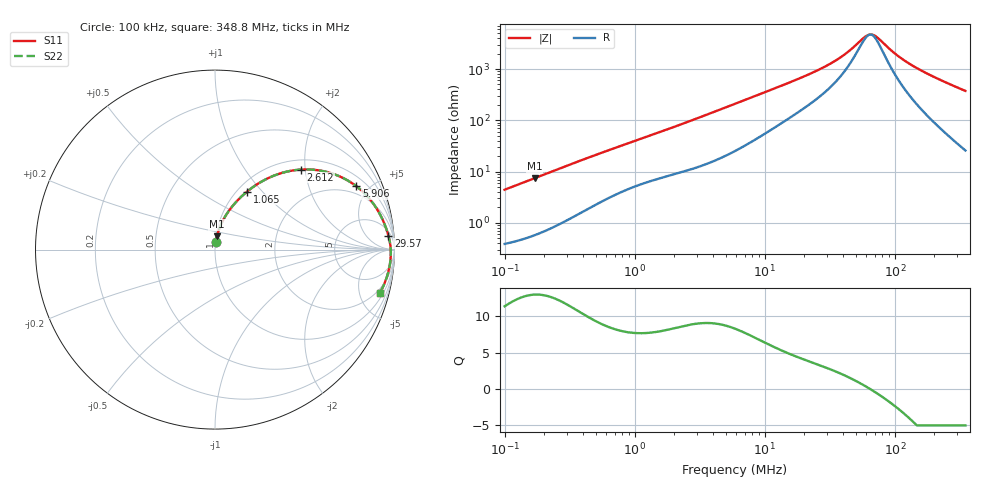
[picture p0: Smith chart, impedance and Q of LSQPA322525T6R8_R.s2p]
! LSQPA322525T6R8_R  S-PARAMETER MODEL  ( General Type )
! Model Generated by TAIYO YUDEN Corporation (http://www.ty-top.com)
! Version 3.0
! TAIYO YUDEN Control No. 110926NF25SB-FKC
! Copyright(c) 2007 TAIYO YUDEN CO.,LTD. All Rights Reserved.
! Product Description (link to TY-COMPAS)
! https://ds.yuden.co.jp/TYCOMPAS/or/detail?pn=LSQPA322525T6R8MR&u=M
! Products Name : Inductors
! Characteristics :
!  Inductance : 6.8 uH , SRF(min) : 50 MHz , DC Resistance(max) : 0.156 Ohm
!  Rated Current : Saturation :950 mA , Temp Rise : 940 mA (40 degC)
!  Case Size : 3.2 x 2.5 / 0.126 x 0.098 [mm/inch] , Thickness : 2.5 / 0.098 [mm/inch]
!  (Conditions: Temperature = 25 degC , DC Bias Current/Voltage = 0A / 0V)
! External Node Assignments :
!  1  o---GGG---o  2
! GND o---------o GND
! Frequency Range : 0.1MHz  -  348.750116MHz  [ 402 STEP ]
# MHz S RI R 50
! Freq[MHz].  S11 Real  S11 Imag  S21 Real  S21 Imag  S12 Real  S12 Imag  S22 Real  S22 Imag
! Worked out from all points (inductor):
!   401 points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, 100 kHz to 348.8 MHz, reference 50 ohm
!   read as one part in series: L = 7 uH near 104.2 kHz
!   highest Q = 12.9 at 169.9 kHz (marker M1), where L = 6.97 uH
!   self-resonance near 64.6 MHz
!   S11 on the Smith chart (normalised r, x): 100 kHz: 1.01, +0.09; 1.065 MHz: 1.11, +0.83; 2.612 MHz: 1.22, +1.89; 5.906 MHz: 1.50, +4.17; 29.57 MHz: 8, +22; 348.8 MHz: 1.52, -7.47
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0.1  0.00581 0.0438  0.9942 -0.0438  0.9942 -0.0438  0.00581 0.0438
0.169927  0.0111 0.0732  0.9889 -0.0732  0.9889 -0.0732  0.0111 0.0732
0.392077  0.0418 0.1577  0.9582 -0.1577  0.9582 -0.1577  0.0418 0.1577
0.666246  0.0949 0.2392  0.9051 -0.2392  0.9051 -0.2392  0.0949 0.2392
1.06495  0.1787 0.3233  0.8213 -0.3233  0.8213 -0.3233  0.1787 0.3233
1.537242  0.2773 0.3887  0.7227 -0.3887  0.7227 -0.3887  0.2773 0.3887
2.612196  0.4779 0.4458  0.5221 -0.4458  0.5221 -0.4458  0.4779 0.4458
3.770673  0.6331 0.4298  0.3669 -0.4298  0.3669 -0.4298  0.6331 0.4298
5.905507  0.788 0.3527  0.212 -0.3527  0.212 -0.3527  0.788 0.3527
10.45281  0.8991 0.2312  0.1009 -0.2312  0.1009 -0.2312  0.8991 0.2312
23.15412  0.9577 0.1062  0.0423 -0.1062  0.0423 -0.1062  0.9577 0.1062
29.57357  0.9662 0.0779  0.0338 -0.0779  0.0338 -0.0779  0.9662 0.0779
40.98306  0.974 0.044  0.026 -0.044  0.026 -0.044  0.974 0.044
57.96438  0.9785 0.0104  0.0215 -0.0104  0.0215 -0.0104  0.9785 0.0104
62.89069  0.9791 0.00257  0.0209 -0.00257  0.0209 -0.00257  0.9791 0.00257
66.85828  0.9794 -0.00332  0.0206 0.00332  0.0206 0.00332  0.9794 -0.00332
71.07618  0.9796 -0.00925  0.0204 0.00925  0.0204 0.00925  0.9796 -0.00925
90.78195  0.9794 -0.0337  0.0206 0.0337  0.0206 0.0337  0.9794 -0.0337
115.9511  0.9774 -0.0603  0.0226 0.0603  0.0226 0.0603  0.9774 -0.0603
154.2634  0.9721 -0.0957  0.0279 0.0957  0.0279 0.0957  0.9721 -0.0957
231.9469  0.9555 -0.1586  0.0445 0.1586  0.0445 0.1586  0.9555 -0.1586
348.7501  0.919 -0.2404  0.081 0.2404  0.081 0.2404  0.919 -0.2404
